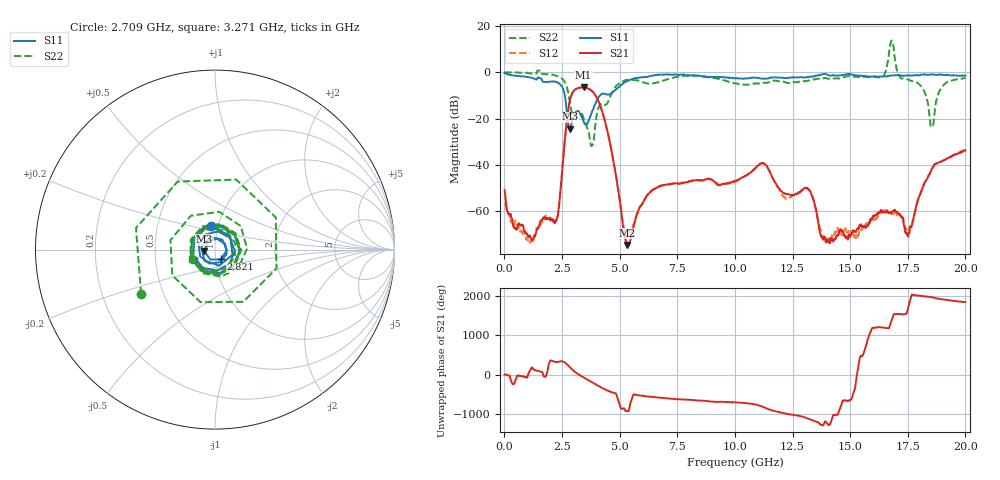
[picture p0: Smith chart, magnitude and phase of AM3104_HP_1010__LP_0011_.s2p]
!Created with skrf (http://scikit-rf.org).
# Hz S RI R 50.0
!freq ReS11 ImS11 ReS21 ImS21 ReS12 ImS12 ReS22 ImS22
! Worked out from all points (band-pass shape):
!   1601 points, 10 MHz to 20 GHz, reference 50 ohm
!   highest |S21| = -6.52 dB at 3.433 GHz (marker M1); lowest = -74.5 dB at 5.332 GHz (marker M2)
!   |S21| within 3 dB of the highest: 2.922 GHz to 3.922 GHz (999.7 MHz wide, 29.2 % of centre)
!   lowest |S11| = -24.4 dB at 2.846 GHz (marker M3), VSWR 1.13, Z = 44.4 - j0.906 ohm
!   |S11| at or under -10 dB: 2.623 GHz to 4.152 GHz (1.529 GHz wide, 45.1 % of centre)
!   |S22| runs from -31.9 to 13.7 dB; largest |S21 - S12| = 0.021
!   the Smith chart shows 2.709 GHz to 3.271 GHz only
!   S11 on the Smith chart (normalised r, x): 2.709 GHz: 0.93, +0.24; 2.821 GHz: 1.06, -0.12; 3.271 GHz: 0.78, -0.09
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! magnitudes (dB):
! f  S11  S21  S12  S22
! 10 MHz  -0.3  -50.8  -56.5  0.0
! 1.134 GHz  -2.3  -71.4  -73.3  -0.5
! 2.221 GHz  -4.1  -64.3  -63.9  -1.4
! 2.709 GHz  -17.7  -20.8  -20.8  -6.4
! 2.821 GHz  -23.9  -13.1  -13.2  -11.9
! 2.846 GHz  -24.4  -12.0  -12.0  -13.5
! 3.271 GHz  -17.6  -6.6  -6.7  -17.0
! 3.346 GHz  -18.9  -6.5  -6.6  -17.5
! 3.433 GHz  -21.1  -6.5  -6.6  -19.8
! 3.796 GHz  -17.1  -8.1  -8.1  -31.8
! 4.32 GHz  -9.3  -19.5  -19.5  -13.9
! 5.332 GHz  -3.8  -74.5  -74.6  -3.3
! 6.682 GHz  -1.1  -49.4  -49.5  -4.3
! 10.01 GHz  -2.7  -47.1  -47.3  -4.8
! 11.2 GHz  -2.8  -39.1  -39.3  -4.6
! 13.34 GHz  -2.0  -53.2  -53.0  -3.3
! 14.03 GHz  -1.2  -73.2  -71.9  -2.7
! 16.68 GHz  -1.5  -60.7  -60.7  7.2
! 17.5 GHz  -1.4  -70.9  -68.6  -3.1
! 18.54 GHz  -0.9  -41.8  -41.9  -23.6
! 19 GHz  -1.2  -38.3  -38.2  -6.2
! 20 GHz  -1.4  -33.6  -33.4  -2.5
